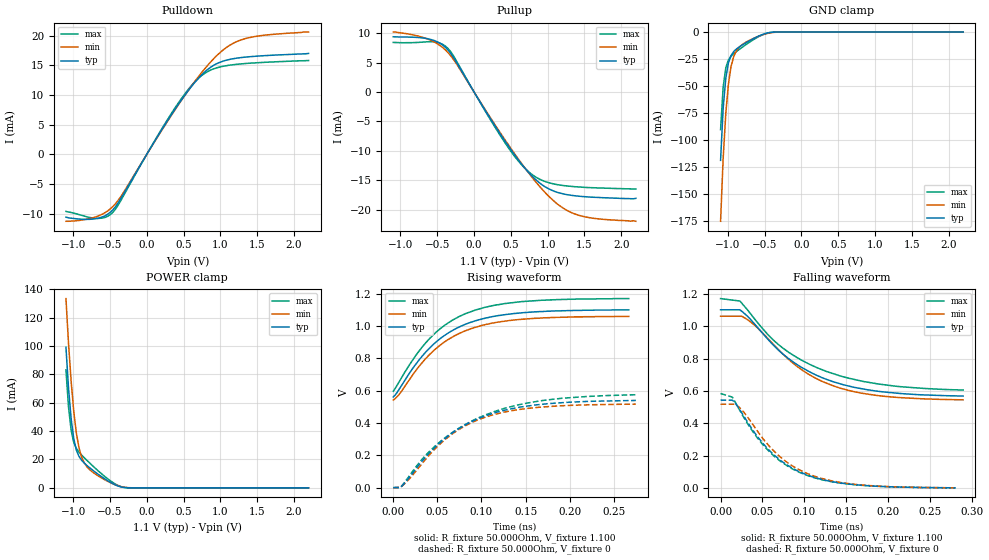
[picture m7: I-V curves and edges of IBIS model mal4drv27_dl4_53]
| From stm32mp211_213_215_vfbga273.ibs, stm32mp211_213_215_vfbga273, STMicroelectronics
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[Model] mal4drv27_dl4_53
Model_type   I/O
Polarity   Non-Inverting
Enable   Active-High
C_comp   1.656pF   1.654pF   1.662pF
C_comp_pullup   832.475fF   825.290fF   839.619fF
C_comp_pulldown 737.556fF   736.745fF   750.731fF
Vinh = 327.000mV
Vinl = 207.000mV
Vmeas = 267.000mV
Vref = 0.00V
Rref = 50Ohms
Cref = 0pF
[Model Spec]
Vinh   327.000mV   317.000mV   344.000mV
Vinl   207.000mV   197.000mV   224.000mV
Vmeas   267.000mV   257.000mV   284.000mV
Vref   0.00V   0.00V   0.00V
D_overshoot_ampl_h 0.3 NA   NA
D_overshoot_ampl_l 0.3 NA   NA
D_overshoot_area_l 100.000m NA   NA
D_overshoot_area_h 100.000m NA   NA
[Receiver Thresholds]
Vth = 267.000mV
Vth_min = 257.000mV
Vth_max = 284.000mV
Vinh_ac = 600.000mV
Vinh_dc = 600.000mV
Vinl_ac = -600.000mV
Vinl_dc = -600.000mV
Tslew_ac = 5.000ns
Threshold_sensitivity = 0.5
Reference_supply Pullup_ref
[Temperature Range]   25.000   125.000   -40.000
[Voltage Range]   1.100V   1.060V   1.170V
[GND Clamp Reference]   0.00V   0.00V   0.00V
[C Comp Corner]
| variable   typ   min   max
C_comp 1.662pF   1.656pF   1.654pF
C_comp_pullup 832.475fF   839.619fF   825.290fF
C_comp_pulldown 736.745fF   750.731fF   737.556fF
[Pulldown Reference]   0.00V   0.00V   0.00V
[POWER Clamp Reference]   1.100V   1.060V   1.170V
[Pullup Reference]   1.100V   1.060V   1.170V
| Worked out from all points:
|   slope of the pulldown table from 0 to 0.165 V, typ, clamps not added: 49 ohm
|   slope of the pullup table from 0 to 0.165 V, typ, clamps not added: 48.8 ohm
|   GND clamp passes 1 mA (typ) near -0.47 V on its own axis
|   POWER clamp passes 1 mA (typ) near -0.37 V on its own axis
|   rising waveform, R_fixture 50.000Ohm, V_fixture 1.100: 20-80 % time 60.3ps typ, 60.1ps min, 60.7ps max; typ from 0.56 V to 1.1 V
|   rising waveform, R_fixture 50.000Ohm, V_fixture 0: 20-80 % time 73.9ps typ, 67.6ps min, 85.1ps max; typ from 0 V to 0.539 V
|   falling waveform, R_fixture 50.000Ohm, V_fixture 1.100: 20-80 % time 80.9ps typ, 76ps min, 88.9ps max; typ from 1.1 V to 0.568 V
|   falling waveform, R_fixture 50.000Ohm, V_fixture 0: 20-80 % time 61.6ps typ, 61.5ps min, 61.8ps max; typ from 0.543 V to 0.001 V
[GND Clamp]
-1.099V   -119mA     -175.5mA   -90.46mA
-1.064V   -70.81mA   -117.3mA   -51.1mA
-1.028V   -42.76mA   -75.52mA   -33.21mA
-992.7mV  -28.64mA   -48.36mA   -25.94mA
-957.3mV  -21.83mA   -32.18mA   -22.47mA
-921.8mV  -18.22mA   -22.95mA   -20.16mA
-886.4mV  -15.9mA    -17.64mA   -18.21mA
-815.5mV  -12.5mA    -12.17mA   -14.62mA
-567.3mV  -3.324mA   -3.512mA   -3.774mA
-460.9mV  -879.1uA   -1.269mA   -863.6uA
-390mV    -181.5uA   -432.7uA   -123.2uA
2.198V    31.48nA    451.7nA    3.508nA
[Power Clamp]
-1.098V   99.1mA     133.3mA    83.09mA
-1.063V   70.06mA    101.6mA    56.85mA
-1.027V   48.48mA    74.82mA    40.4mA
-991.8mV  34.54mA    53.74mA    31.95mA
-956.4mV  26.58mA    38.45mA    27.74mA
-920.9mV  22.17mA    28.22mA    25.15mA
-885.5mV  19.46mA    21.74mA    23.1mA
-814.5mV  15.82mA    14.94mA    19.43mA
-743.6mV  12.83mA    11.41mA    15.93mA
-460mV    2.904mA    2.84mA     3.733mA
-282.7mV  117.7uA    274uA      108uA
2.199V    -10.68nA   -391.6nA   -2.283nA
[Pulldown]
-1.099V   -10.6mA    -11.3mA    -9.64mA
-673.6mV  -10.82mA   -10.47mA   -10.82mA
-567.3mV  -10.38mA   -9.838mA   -10.65mA
-460.9mV  -9.361mA   -8.811mA   -9.786mA
-319.1mV  -6.753mA   -6.481mA   -7.043mA
106.4mV   2.186mA    2.129mA    2.27mA
425.4mV   8.356mA    8.267mA    8.584mA
673.6mV   12.42mA    12.62mA    12.48mA
886.4mV   14.82mA    15.81mA    14.29mA
1.099V    15.91mA    18.15mA    14.97mA
1.347V    16.38mA    19.53mA    15.3mA
2.198V    17mA       20.6mA     15.8mA
[Pullup]
-1.098V   9.4mA      10.2mA     8.43mA
-601.8mV  8.981mA    8.865mA    8.547mA
-460mV    8.276mA    7.881mA    8.293mA
-353.6mV  7.142mA    6.699mA    7.406mA
-282.7mV  5.928mA    5.592mA    6.211mA
249.1mV   -5.06mA    -4.895mA   -5.266mA
497.3mV   -9.75mA    -9.542mA   -10.04mA
745.5mV   -13.75mA   -13.82mA   -13.62mA
958.2mV   -16.08mA   -17.01mA   -15.2mA
1.206V    -17.32mA   -19.72mA   -15.91mA
1.419V    -17.73mA   -20.97mA   -16.16mA
2.199V    -18.1mA    -22mA      -16.52mA
[Ramp]
R_load=50.000Ohm
dV/dt_r   323.370mV/69.000ps  310.799mV/65.000ps  345.390mV/75.000ps
dV/dt_f   323.370mV/73.000ps  310.799mV/70.500ps  345.390mV/78.000ps
[Rising waveform]
R_fixture=50.000Ohm
V_fixture=1.100
V_fixture_min=1.060
V_fixture_max=1.170
0s        560.5mV    541.4mV    596mV
9ps       627.8mV    592.5mV    676.5mV
24ps      751.8mV    712.2mV    805.1mV
40ps      856.5mV    816.8mV    914.9mV
59ps      944.3mV    904.3mV    1.007V
81ps      1.008V     968.3mV    1.074V
109ps     1.054V     1.014V     1.121V
146ps     1.081V     1.041V     1.151V
183ps     1.093V     1.052V     1.162V
267ps     1.099V     1.059V     1.169V
[Rising waveform]
R_fixture=50.000Ohm
V_fixture=0
0s        -400.6uV   -2.057mV   -176.4uV
8ps       -400.6uV   1.617mV    -176.4uV
18ps      60.71mV    51.15mV    70.49mV
34ps      172.2mV    157.6mV    183.1mV
57ps      296mV      288.5mV    301mV
77ps      372.9mV    367.7mV    375.7mV
104ps     442.4mV    434.6mV    448.2mV
129ps     482.1mV    470.1mV    494.3mV
168ps     514.9mV    497.9mV    537.6mV
275ps     538.7mV    516mV      573.7mV
[Falling waveform]
R_fixture=50.000Ohm
V_fixture=1.100
V_fixture_min=1.060
V_fixture_max=1.170
0s        1.102V     1.062V     1.171V
23ps      1.102V     1.062V     1.156V
31ps      1.067V     1.045V     1.109V
53ps      940.2mV    943.6mV    968.5mV
73ps      834.7mV    835.1mV    870.8mV
97ps      745.1mV    730.7mV    789.6mV
126ps     672.8mV    649mV      721.6mV
155ps     627.7mV    600.6mV    676.7mV
189ps     597.2mV    570.8mV    643mV
290ps     568.5mV    545.1mV    605.7mV
[Falling waveform]
R_fixture=50.000Ohm
V_fixture=0
0s        543.3mV    517.9mV    584mV
14ps      543.3mV    517.9mV    562.1mV
21ps      499.9mV    504.8mV    497.8mV
39ps      354.3mV    388.5mV    345.2mV
57ps      239mV      265.6mV    231.4mV
79ps      144mV      160.2mV    138.7mV
101ps     85.09mV    95.29mV    82.25mV
130ps     42.3mV     47.29mV    41.32mV
166ps     17.6mV     19.72mV    17.49mV
281ps     1.066mV    1.245mV    1.034mV
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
